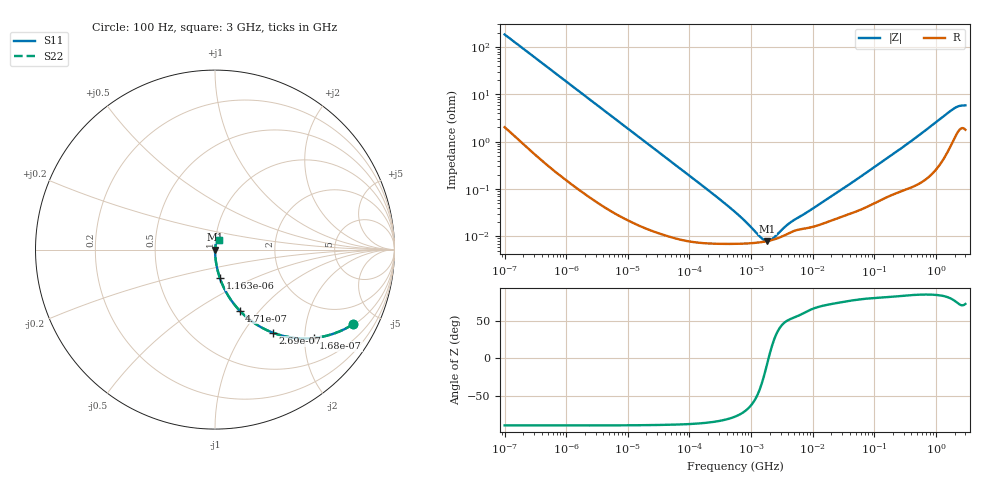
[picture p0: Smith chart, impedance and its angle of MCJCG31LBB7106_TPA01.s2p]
! MCJCG31LBB7106_TPA01  S-PARAMETER MODEL  ( Standard Model )
! Model Generated by TAIYO YUDEN Corporation (http://www.ty-top.com)
! Version 1.0
! TAIYO YUDEN Control No. 220601
! Copyright(c) 2015 TAIYO YUDEN CO.,LTD. All Rights Reserved.
! Product Description (link to TY-COMPAS)
! https://ds.yuden.co.jp/TYCOMPAS/or/detail?pn=MCJCG31LBB7106KTPA01&u=M
! Products Name : Multilayer Ceramic Capacitors
! Characteristics :
!  Capacitance : 10 [uF] , Rated Voltage : 35 [V] , TCC : X7R
!  Case Size : 3.2 x 1.6 / 0.126 x 0.063 [mm/inch] , Thickness : 1.6 / 0.063 [mm/inch]
!  (Conditions: Temperature = 25 [degC] , DC Bias Voltage = 0 [V])
! External Node Assignments :
!  1  o---| |---o  2
! GND o---------o GND
! Frequency Range : 100Hz  -  3GHz  [ 401 STEP ]
# MHZ S RI R 50
! Freq[MHz].  S11 Real  S11 Imag  S21 Real  S21 Imag  S12 Real  S12 Imag  S22 Real  S22 Imag
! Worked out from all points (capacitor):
!   401 points, 100 Hz to 3 GHz, reference 50 ohm
!   read as one part in series: C = 8.61 uF near 109 Hz
!   lowest |Z| = 7.98 mohm at 1.828 MHz (marker M1)
!   series resonance near 1.92 MHz, so ESL is about 800 pH
!   S11 on the Smith chart (normalised r, x): 100 Hz: 1.04, -3.69; 168 Hz: 1.02, -2.21; 269 Hz: 1.01, -1.38; 471 Hz: 1.01, -0.79; 1.163 kHz: 1.00, -0.32; 3 GHz: 1.04, +0.11
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0.0001  0.7704 -0.4151  0.2296 0.4151  0.2296 0.4151  0.7704 -0.4151
0.000168  0.5492 -0.4926  0.4508 0.4926  0.4508 0.4926  0.5492 -0.4926
0.000269  0.3241 -0.4635  0.6759 0.4635  0.6759 0.4635  0.3241 -0.4635
0.000471  0.1374 -0.34  0.8626 0.34  0.8626 0.34  0.1374 -0.34
0.000724  0.064 -0.2407  0.936 0.2407  0.936 0.2407  0.064 -0.2407
0.001163  0.0264 -0.1564  0.9736 0.1564  0.9736 0.1564  0.0264 -0.1564
0.001788  0.0117 -0.1035  0.9883 0.1035  0.9883 0.1035  0.0117 -0.1035
0.005476  0.00151 -0.0343  0.9985 0.0343  0.9985 0.0343  0.00151 -0.0343
0.031977  0.000151 -0.00594  0.9998 0.00594  0.9998 0.00594  0.000151 -0.00594
0.221826  7.1e-05 -0.000852  0.9999 0.000852  0.9999 0.000852  7.1e-05 -0.000852
0.547723  6.94e-05 -0.000321  0.9999 0.000321  0.9999 0.000321  6.94e-05 -0.000321
1.295438  7.38e-05 -7.95e-05  0.9999 7.95e-05  0.9999 7.95e-05  7.38e-05 -7.95e-05
1.473992  7.55e-05 -5.24e-05  0.9999 5.24e-05  0.9999 5.24e-05  7.55e-05 -5.24e-05
1.827928  7.92e-05 -9.57e-06  0.9999 9.57e-06  0.9999 9.57e-06  7.92e-05 -9.57e-06
2.266852  8.48e-05 3.2e-05  0.9999 -3.2e-05  0.9999 -3.2e-05  8.48e-05 3.2e-05
2.579298  8.93e-05 5.68e-05  0.9999 -5.68e-05  0.9999 -5.68e-05  8.93e-05 5.68e-05
4.323298  0.000121 0.000155  0.9999 -0.000155  0.9999 -0.000155  0.000121 0.000155
9.794414  0.000157 0.000345  0.9998 -0.000345  0.9998 -0.000345  0.000157 0.000345
175.1444  0.000731 0.00477  0.9993 -0.00477  0.9993 -0.00477  0.000731 0.00477
1868.531  0.012 0.0462  0.988 -0.0462  0.988 -0.0462  0.012 0.0462
2317.205  0.0192 0.0517  0.9808 -0.0517  0.9808 -0.0517  0.0192 0.0517
3000  0.0205 0.0537  0.9795 -0.0537  0.9795 -0.0537  0.0205 0.0537
